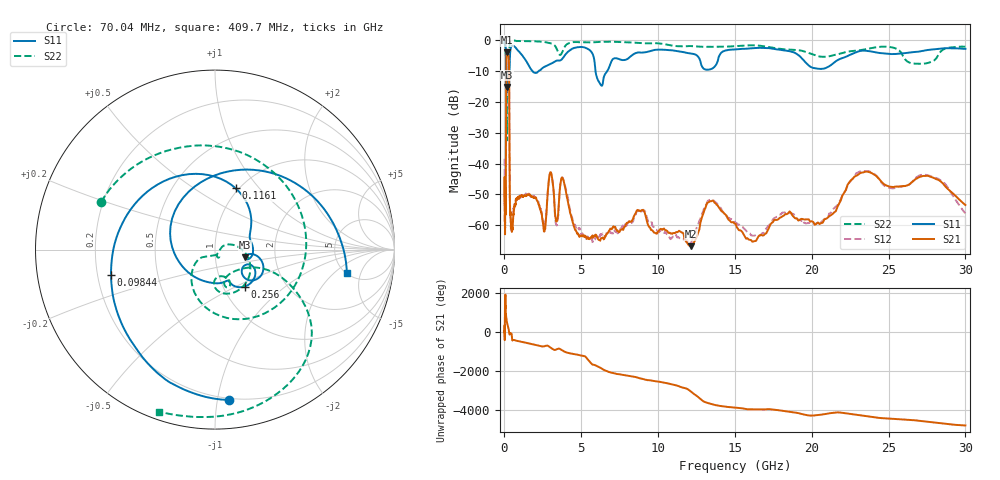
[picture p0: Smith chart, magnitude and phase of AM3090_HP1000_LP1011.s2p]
! Date/Time: Thu, Feb 28, 2019 2:02 PM
! Network Analyzer: Agilent Technologies E8364B Rev: A.07.50.67
! Sweep from 0.010 to 30.000 GHz, 1601 Points, Sweep Type: LOG
! Power Supply: 5.023 V, 0.002 A
# Hz S DB R 50
!freq MagS11 AngS11 MagS21 AngS21 MagS12 AngS12 MagS22 AngS22
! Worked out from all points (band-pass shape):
!   1601 points, 10 MHz to 30 GHz, reference 50 ohm
!   highest |S21| = -3.98 dB at 169.8 MHz (marker M1); lowest = -66.8 dB at 12.13 GHz (marker M2)
!   |S21| within 3 dB of the highest: 123 MHz to 287.5 MHz (164.5 MHz wide, 80.2 % of centre)
!   lowest |S11| = -15.2 dB at 154.4 MHz (marker M3), VSWR 1.42, Z = 70 - j5.86 ohm
!   |S11| at or under -10 dB: 118.2 MHz to 326.2 MHz (208 MHz wide, 93.6 % of centre); 1.81 GHz to 2.239 GHz (429.6 MHz wide, 21.2 % of centre); 5.925 GHz to 6.696 GHz (770.8 MHz wide, 12.2 % of centre)
!   |S22| runs from -32.5 to -0.2 dB; largest |S21 - S12| = 0.013
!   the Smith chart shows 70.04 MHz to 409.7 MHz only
!   S11 on the Smith chart (normalised r, x): 70.04 MHz: 0.19, -1.08; 98.44 MHz: 0.26, -0.11; 116.1 MHz: 0.97, +0.76; 256 MHz: 1.26, -0.56; 409.7 MHz: 5.07, -2.97
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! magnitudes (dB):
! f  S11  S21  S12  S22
! 10 MHz  -0.3  -52.1  -38.5  -0.7
! 38.04 MHz  -0.5  -60.5  -58.0  -1.6
! 70.04 MHz  -1.5  -52.4  -52.6  -3.3
! 84.71 MHz  -2.5  -52.6  -50.5  -4.7
! 98.44 MHz  -4.5  -34.9  -35.2  -5.7
! 116.1 MHz  -8.9  -11.2  -11.2  -10.9
! 144.7 MHz  -14.2  -4.4  -4.4  -32.5
! 154.4 MHz  -15.2  -4.1  -4.1  -24.6
! 169.8 MHz  -12.6  -4.0  -3.9  -14.4
! 256 MHz  -11.6  -4.9  -4.8  -13.1
! 299 MHz  -14.6  -9.6  -9.5  -10.7
! 350.9 MHz  -5.7  -51.6  -50.3  -0.9
! 409.7 MHz  -2.5  -58.1  -60.4  -0.4
! 550.5 MHz  -1.9  -58.6  -57.9  -0.3
! 2.084 GHz  -10.6  -51.7  -51.2  -0.5
! 3.002 GHz  -7.7  -42.9  -42.8  -1.1
! 7.926 GHz  -6.3  -59.5  -60.2  -0.7
! 12.13 GHz  -4.4  -66.8  -65.9  -2.0
! 13.47 GHz  -9.4  -52.2  -51.7  -2.2
! 20.2 GHz  -9.1  -59.8  -59.8  -4.9
! 23.36 GHz  -3.4  -42.9  -42.6  -3.1
! 30 GHz  -2.9  -53.4  -56.1  -2.2
